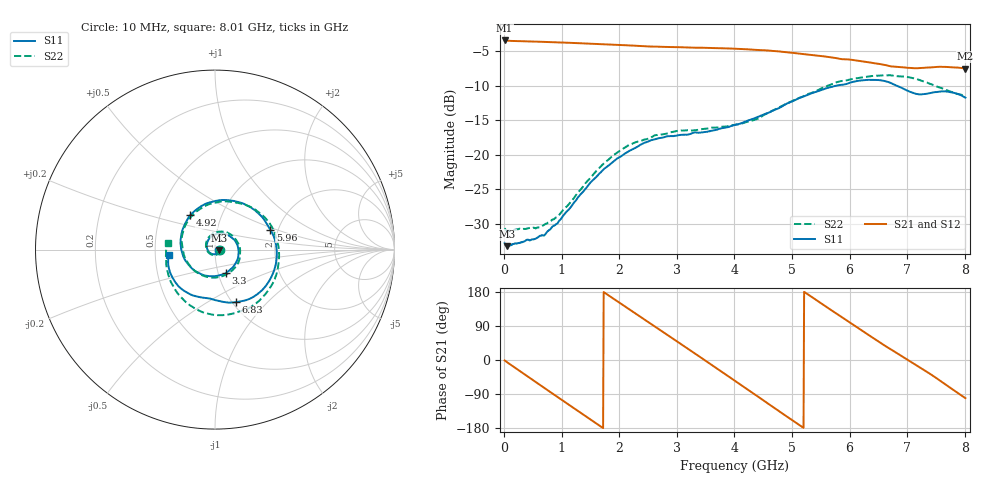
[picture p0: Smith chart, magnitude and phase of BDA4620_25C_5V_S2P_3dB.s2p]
!Agilent Technologies,E5071B,MY42404982,A.09.10
!Date: Wed May 06 08:58:43 2026
!Data & Calibration Information:
!Freq	S11:SOLT2(ON)	S21:SOLT2(ON)	S12:SOLT2(ON)	S22:SOLT2(ON)
# Hz S RI R 50
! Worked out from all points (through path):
!   801 points, 10 MHz to 8.01 GHz, reference 50 ohm
!   highest |S21| = -3.44 dB at 10 MHz (marker M1); lowest = -7.5 dB at 8.01 GHz (marker M2)
!   group delay of S21, straight-line fit = 285 ps
!   lowest |S11| = -33.2 dB at 60 MHz (marker M3), VSWR 1.04, Z = 52.2 - j0.309 ohm
!   |S11| at or under -10 dB: start of sweep to 5.761 GHz; 6.821 GHz to end of sweep
!   |S22| runs from -31.0 to -8.5 dB; largest |S21 - S12| = 0.0031
!   S11 on the Smith chart (normalised r, x): 10 MHz: 1.05, -0.00; 3.3 GHz: 1.09, -0.29; 4.92 GHz: 0.71, +0.29; 5.96 GHz: 1.82, +0.45; 6.83 GHz: 1.04, -0.67; 8.01 GHz: 0.59, -0.04
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1e7  0.0229 -0.0016  0.6725 -0.0144  0.6734 -0.0146  0.0294 -0.00201
6e7  0.0217 -0.00296  0.6654 -0.077  0.6671 -0.0781  0.028 -0.00374
3.6e8  0.0171 -0.0165  0.5218 -0.4094  0.5224 -0.4106  0.0212 -0.0201
7.3e8  -0.00666 -0.0264  0.149 -0.6391  0.1488 -0.64  -0.00675 -0.0311
1.03e9  -0.0341 -0.0128  -0.2021 -0.6169  -0.2029 -0.6177  -0.0371 -0.0153
1.35e9  -0.0461 0.0261  -0.5019 -0.3998  -0.5022 -0.4003  -0.0505 0.0275
1.64e9  -0.0266 0.067  -0.6264 -0.0944  -0.6275 -0.0947  -0.0311 0.0729
1.93e9  0.02 0.0896  -0.5826 0.2273  -0.5836 0.2282  0.0194 0.0996
2.32e9  0.0934 0.067  -0.2934 0.5402  -0.2945 0.5408  0.0998 0.075
2.68e9  0.1319 -0.00485  0.0847 0.5997  0.0854 0.6008  0.1395 0.00355
3.3e9  0.0606 -0.1319  0.5643 0.1894  0.5656 0.1893  0.0743 -0.1313
3.64e9  -0.0246 -0.1487  0.5684 -0.1685  0.5685 -0.1698  -0.0199 -0.1563
4.01e9  -0.1224 -0.1099  0.3358 -0.4805  0.3354 -0.4816  -0.1255 -0.107
4.46e9  -0.1909 0.0203  -0.1191 -0.5612  -0.1197 -0.5614  -0.1845 0.0372
4.92e9  -0.1378 0.1914  -0.4792 -0.2743  -0.4798 -0.2747  -0.1013 0.2139
5.35e9  0.0457 0.2764  -0.51 0.1317  -0.5104 0.1322  0.0958 0.2654
5.96e9  0.3081 0.1115  -0.116 0.4771  -0.116 0.478  0.3412 0.0644
6.31e9  0.3358 -0.0945  0.1756 0.435  0.177 0.4354  0.3425 -0.1351
6.68e9  0.1946 -0.2736  0.3763 0.2288  0.3777 0.2285  0.2086 -0.314
6.83e9  0.1146 -0.2934  0.4132 0.1299  0.4144 0.1294  0.1246 -0.3485
7.38e9  -0.0915 -0.2638  0.3518 -0.2458  0.3521 -0.247  -0.1799 -0.2745
8.01e9  -0.2575 -0.0313  -0.0779 -0.4143  -0.0786 -0.4157  -0.2645 0.0367
